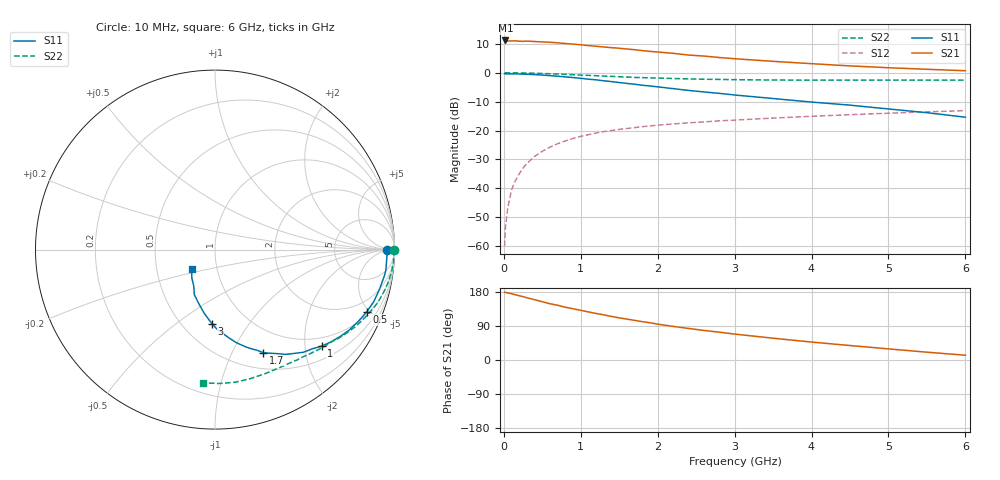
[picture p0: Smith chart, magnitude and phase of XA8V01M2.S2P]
! SIEMENS Discrete & RF Semiconductors
! BFY180
! Si NPN RF Bipolar Junction Transistor in MICRO-X
! VCE = 8 V  IC = 1.2 mA
! Common Emitter S-Parameters:  May  1997
# GHz  S  MA  R  50
!  f  S11  S21  S12  S22
! GHz  MAG  ANG  MAG  ANG  MAG  ANG  MAG  ANG
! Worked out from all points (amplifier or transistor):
!   36 points, 10 MHz to 6 GHz, reference 50 ohm
!   highest |S21| = 11.2 dB at 20 MHz (marker M1)
!   |S21| within 3 dB of that: start of sweep to 1.613 GHz
!   unconditionally stable (mu >= 1): 3.958 GHz to end of sweep
!   at 250 MHz: K = 0.09, MSG = 21.9 dB, |S12| = -33.0 dB
!   at 1.4 GHz: K = 0.51, MSG = 14.3 dB, |S12| = -20.0 dB
!   at 6 GHz: K = 1.05, MAG = 5.6 dB, |S12| = -13.1 dB
!   S11 on the Smith chart (normalised r, x): 10 MHz: 49, -4; 500 MHz: 1.15, -4.79; 1 GHz: 0.79, -2.37; 1.7 GHz: 0.69, -1.33; 3 GHz: 0.69, -0.68; 6 GHz: 0.75, -0.17
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0.01  0.9606 -0.2  3.562 178.9  0.001 88.4  0.9959 -0.2
0.02  0.9557 -1.0  3.624 178.3  0.0021 97.7  0.9999 -0.5
0.05  0.9588 -2.0  3.554 177.3  0.0045 82.7  0.9968 -1.4
0.1  0.958 -4.6  3.548 174.9  0.0094 90.1  0.9961 -2.8
0.15  0.9591 -7.0  3.577 172.2  0.0136 85.6  0.997 -4.1
0.25  0.9473 -11.5  3.495 167.2  0.0225 82.0  0.9921 -6.9
0.3  0.9426 -13.6  3.534 164.2  0.0269 80.3  0.988 -8.2
0.5  0.913 -22.4  3.42 153.8  0.0438 74.5  0.9717 -13.5
0.6  0.8927 -26.7  3.371 148.4  0.0518 71.7  0.9621 -15.9
0.8  0.8494 -34.7  3.208 139.2  0.0662 66.0  0.9381 -20.7
1  0.8012 -42.2  3.047 131.0  0.0795 61.2  0.9132 -25.1
1.1  0.7744 -45.5  2.95 126.9  0.085 59.0  0.9015 -27.1
1.5  0.6778 -58.8  2.657 111.2  0.1047 50.9  0.8539 -34.6
1.7  0.6343 -64.9  2.506 104.6  0.1125 48.0  0.8307 -37.8
2  0.5705 -72.2  2.288 94.6  0.1241 43.9  0.8099 -42.4
2.2  0.532 -77.1  2.171 88.7  0.1302 41.2  0.7957 -45.3
2.6  0.4657 -85.1  1.947 78.0  0.1413 37.3  0.7729 -50.6
3  0.4126 -92.5  1.75 68.4  0.1517 33.5  0.7594 -55.6
3.5  0.3585 -99.8  1.577 57.5  0.1644 29.6  0.7491 -61.8
4.5  0.2755 -114.8  1.315 38.2  0.1883 21.8  0.7454 -74.6
5.5  0.2039 -129.3  1.149 20.6  0.2108 14.1  0.7467 -88.1
6  0.1704 -139.9  1.085 12.6  0.2211 9.8  0.7449 -95.0
